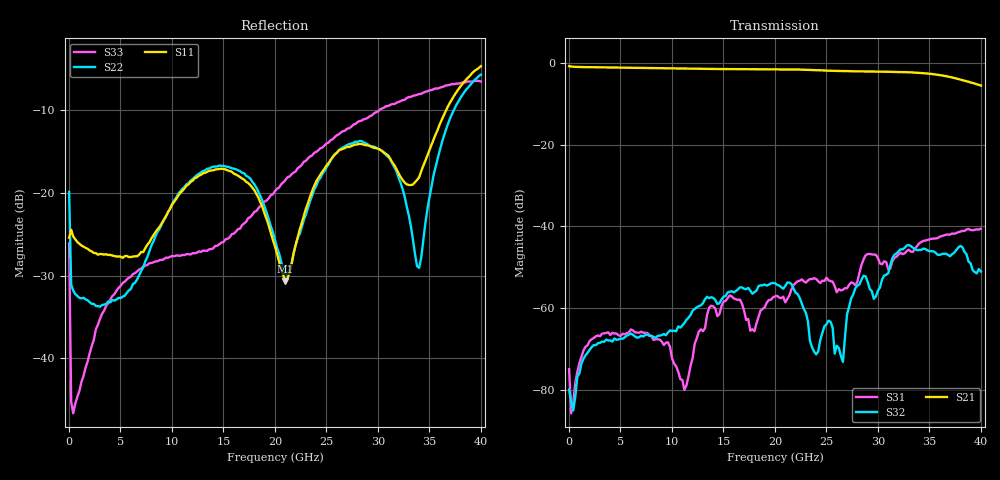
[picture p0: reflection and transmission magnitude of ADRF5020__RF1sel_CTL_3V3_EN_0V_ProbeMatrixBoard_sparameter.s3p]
! Device:  ADRF5020
! Description: SOI MMIC SPDT Non-Reflective Switch
! Frequency:  0.1 -  30 GHz
! Ports:
! 	RFC	= Port 1
!	RF1	= Port 2
!	RF2	= Port 3
! Vdd:  +3.3 Volt
! Vss:  -2.5 Volt
! Control:  0/+3.3 Volt
! State:  RF1 Selected (Vctl= +3.3 V, Ven= 0 V)
! Data:  The device was measured using G-S-G Probes on a matrix board.
!  Data was collected using an calibrated 4 port network analyzer.
!  The reference plane is the package pins of ADRF5020 switch.
! Note:  Analog Devices supplies this data as a sample of measured data at the package pin
!  for this product.  Your particular data for this product may vary.
!  Data was taken at 25 degrees C.
!  Analog Devices reserves the right to change this data at anytime.
# GHZ S DB R 50.0
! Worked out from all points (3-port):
!   201 points, 10 MHz to 40.01 GHz, reference 50 ohm
!   strongest paths, dB at 10 MHz, 10.01 GHz, 20.01 GHz, 30.01 GHz, 40.01 GHz:
!     S21: -0.7, -1.2, -1.5, -2.0, -5.4
!     S32: -80.0, -65.6, -53.9, -55.7, -51.0
!     S31: -75.0, -72.4, -57.1, -47.7, -40.5
!   lowest |S11| = -30.7 dB at 21.01 GHz (marker M1), VSWR 1.06, Z = 51.1 - j2.75 ohm
!   |S11| at or under -10 dB: start of sweep to 36.63 GHz
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0.01  -25.43 72.5  -0.69 0.2  -83.31 -5.8
      -0.69 -0.1  -19.87 70.7  -81.61 -23.2
      -75.00 38.0  -79.99 6.3  -26.11 -51.1
0.41  -25.28 -17.6  -0.83 -5.5  -82.14 68.0
      -0.83 -5.5  -31.83 -22.4  -86.32 63.0
      -82.95 74.3  -85.12 29.7  -46.70 56.8
8.61  -24.39 -42.9  -1.19 -100.5  -67.99 14.9
      -1.19 -100.5  -24.67 -42.0  -66.86 -49.1
      -67.65 13.9  -66.82 -49.8  -28.27 -70.9
11.21  -19.43 -50.4  -1.28 -130.5  -80.08 -31.4
       -1.28 -130.5  -19.27 -58.1  -63.76 -99.5
       -80.08 -36.9  -63.64 -101.4  -27.53 -70.5
20.01  -26.48 -103.0  -1.45 126.6  -57.14 119.1
       -1.46 126.7  -25.72 -127.0  -53.99 66.0
       -57.12 118.5  -53.92 65.9  -19.77 -37.0
21.01  -30.67 -66.6  -1.48 114.5  -58.50 116.5
       -1.48 114.6  -29.77 -92.0  -54.53 57.0
       -58.61 116.9  -54.59 56.8  -18.45 -37.8
26.61  -14.65 -39.7  -1.89 46.7  -55.30 106.4
       -1.89 46.8  -14.47 -61.7  -71.44 -59.8
       -55.51 106.4  -73.21 -39.1  -12.51 -49.5
30.21  -14.75 -67.1  -2.02 1.8  -49.04 89.2
       -2.03 2.0  -14.75 -98.0  -54.77 143.4
       -49.08 89.2  -54.94 143.1  -9.87 -65.2
34.01  -18.09 -32.8  -2.33 -49.5  -44.19 96.8
       -2.33 -49.3  -29.07 -55.2  -45.77 69.6
       -44.15 97.2  -45.74 69.7  -8.00 -81.4
40.01  -4.63 -59.4  -5.43 -134.0  -40.49 40.7
       -5.44 -133.7  -5.66 -55.0  -51.08 22.4
       -40.54 41.3  -51.05 22.0  -6.49 -112.7
